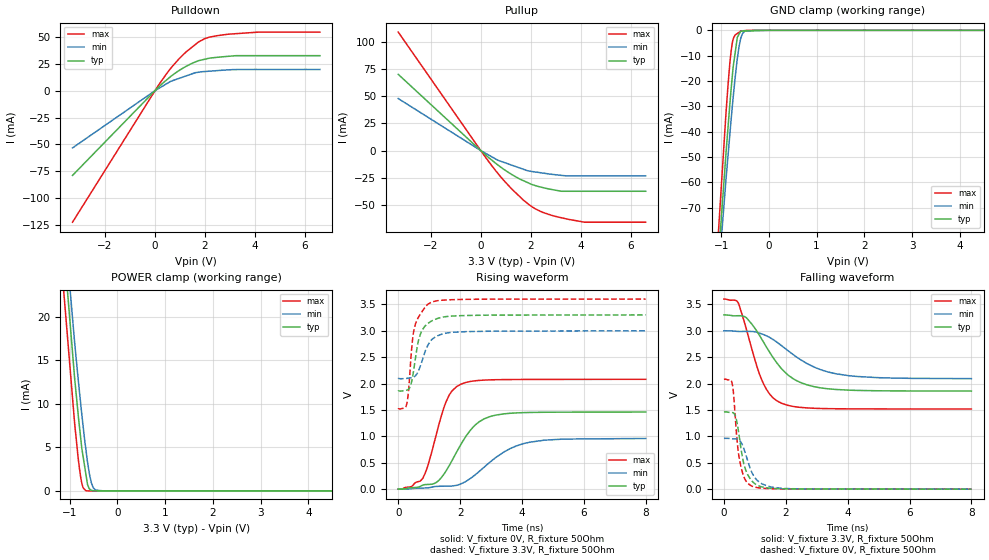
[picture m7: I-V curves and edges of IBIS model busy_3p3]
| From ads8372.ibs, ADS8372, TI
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|   busy_3p3 Model
[Model]   busy_3p3
Model_type   3-state
Polarity   Non-Inverting
Vmeas = 1.65
Vref = 1.65
Cref = 10pF
Rref = 50
|   typ   min   max
|   (nom PVT)   (fast PVT)   (slow PVT)
|C_comp from frequency sweep method (F=1MHz)
|C_comp   3.458e-12   3.339e-12   3.651e-12
|ON state : BUFFER OUTPUT TURNED HIGH
|C_comp   3.458e-12   3.339e-12   3.651e-12
|OFF state: BUFFER IN HIGH IMPEDANCE
|C_comp   2.977e-12   2.823e-12   3.114e-12
|C_comp from LC tank measurement(L=1nH)
|Resonant Frequency(Hz)   5.970e+09   6.100e+09   5.800e+09
|C_comp   7.114e-13   6.814e-13   7.537e-13
|ON state : BUFFER OUTPUT TURNED HIGH
|Resonant Frequency(Hz)   5.970e+09   6.100e+09   5.800e+09
|C_comp   7.114e-13   6.814e-13   7.537e-13
|OFF state: BUFFER IN HIGH IMPEDANCE
|Resonant Frequency(Hz)   6.040e+09   6.210e+09   5.850e+09
C_comp   6.950e-13   6.575e-13   7.409e-13
| Where nom  PVT is Nominal Process, 3.3V, 35C
|   Fast PVT is Strong Process,  3.6V, -40C
|   Slow PVT is Weak Process,   3V, 95C
[Voltage Range]   3.3   3   3.6
|Ambient Temperature   25   85   -40
|Junction Temperature
[Temperature Range]   35   95   -40
[Pullup Reference]   3.3   3   3.6
[Pulldown Reference]   0   0   0
[Power Clamp Reference]   3.3   3   3.6
[GND Clamp Reference]   0   0   0
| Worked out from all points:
|   slope of the pulldown table from 0 to 0.495 V, typ, clamps not added: 46.6 ohm
|   slope of the pullup table from 0 to 0.495 V, typ, clamps not added: 50.7 ohm
|   GND clamp passes 1 mA (typ) near -0.61 V on its own axis
|   POWER clamp passes 1 mA (typ) near -0.63 V on its own axis
|   falling waveform, V_fixture 3.3V, R_fixture 50Ohm: 20-80 % time 1.06ns typ, 1.45ns min, 683ps max; typ from 3.3 V to 1.86 V
|   rising waveform, V_fixture 0V, R_fixture 50Ohm: 20-80 % time 924ps typ, 1.31ns min, 613ps max; typ from 0 V to 1.46 V
|   rising waveform, V_fixture 3.3V, R_fixture 50Ohm: 20-80 % time 304ps typ, 384ps min, 252ps max; typ from 1.86 V to 3.3 V
|   falling waveform, V_fixture 0V, R_fixture 50Ohm: 20-80 % time 304ps typ, 391ps min, 225ps max; typ from 1.46 V to 0.001 V
[Pulldown]
|   Voltage   I(typ)   I(min)   I(max)
-3.3V     -78.98mA   -53.36mA   -122.6mA
176.4mV   4.073mA    2.487mA    6.361mA
633mV     13.32mA    8.781mA    20.94mA
939.6mV   18.45mA    11.28mA    29.19mA
1.246V    22.71mA    13.78mA    36.21mA
1.706V    27.67mA    17.1mA     44.83mA
2.153V    30.2mA     18.15mA    49.79mA
2.934V    32.05mA    19.43mA    52.68mA
4.162V    32.65mA    19.81mA    54.64mA
6.6V      32.65mA    19.81mA    54.64mA
[GND Clamp]
|   Voltage   I(typ)   I(min)   I(max)
-3.3V     -761.3mA   -676.6mA   -965.4mA
-1.115V   -105.4mA   -111.1mA   -97.09mA
-897.6mV  -48.4mA    -58.78mA   -32.56mA
-856.8mV  -38.65mA   -49.79mA   -21.97mA
-792mV    -23.53mA   -35.54mA   -8.421mA
-766.8mV  -18.32mA   -30.35mA   -5.108mA
-738mV    -13.14mA   -24.6mA    -2.94mA
-660mV    -2.733mA   -11.06mA   -1.235mA
-586.8mV  -322.6uA   -3.017mA   -267.8uA
-510mV    -258uA     -378.2uA   -130.5uA
-285mV    -143.4uA   -450.4nA   -1.904uA
6.6V      0A         0A         0A
[Pullup]
|   Voltage   I(typ)   I(min)   I(max)
-3.3V     69.99mA    47.77mA    108.8mA
18mV      -371.7uA   -256.6uA   -591.9uA
478.8mV   -9.46mA    -6.234mA   -15.01mA
708mV     -13.64mA   -9.093mA   -21.59mA
1.246V    -22.07mA   -13.46mA   -35.43mA
1.89V     -29.57mA   -18.59mA   -48.96mA
2.167V    -32.08mA   -19.64mA   -53.36mA
2.473V    -33.96mA   -20.65mA   -56.75mA
2.812V    -35.67mA   -21.75mA   -59.36mA
3.241V    -37.41mA   -22.85mA   -61.83mA
4.151V    -37.41mA   -23.24mA   -65.82mA
6.6V      -37.41mA   -23.24mA   -65.82mA
[POWER Clamp]
|   Voltage   I(typ)   I(min)   I(max)
-3.3V     298.8mA    244.5mA    432.6mA
-1.156V   30.27mA    33.59mA    24.98mA
-897.6mV  13.01mA    17.12mA    7.827mA
-824.4mV  8.877mA    12.96mA    3.87mA
-766.8mV  5.928mA    9.871mA    1.482mA
-720mV    3.976mA    7.457mA    365.5uA
-662.4mV  1.972mA    4.822mA    28.47uA
-627mV    740.4uA    3.325mA    5.896uA
-549mV    64.5uA     984.1uA    3.448uA
-510mV    36.68uA    395.6uA    2.223uA
-462mV    2.437uA    102.5uA    716.8nA
6.6V      0A         0A         0A
[Ramp]
R_load = 50
|   typ   min   max
dV/dt_r   0.876214/9.23938e-10   0.576036/1.31035e-09   1.24786/6.12367e-10
dV/dt_f   0.864611/1.06042e-09   0.543659/1.44481e-09   1.2486/6.81788e-10
[Falling Waveform]
V_fixture = 3.3V
V_fixture_min = 3V
V_fixture_max = 3.6V
R_fixture = 50Ohm
|   Time   V(typ)   V(min)   V(max)
0s        3.3V       3V         3.6V
464ps     3.286V     2.988V     3.528V
724ps     3.249V     2.99V      3.034V
1.02ns    3.032V     2.979V     2.413V
1.228ns   2.836V     2.94V      2.062V
1.518ns   2.556V     2.86V      1.774V
1.86ns    2.283V     2.72V      1.628V
2.444ns   2.029V     2.465V     1.551V
3.62ns    1.889V     2.186V     1.523V
7.998ns   1.859V     2.094V     1.519V
[Rising Waveform]
V_fixture = 0V
V_fixture_min = 0V
V_fixture_max = 0V
R_fixture = 50Ohm
|   Time   V(typ)   V(min)   V(max)
0s        1.371nV    3.229nV    1.196nV
794ps     76.83mV    21.38mV    206.9mV
970ps     89.68mV    25.69mV    469.8mV
1.24ns    131.7mV    52.31mV    1.056V
1.548ns   347.7mV    56.8mV     1.656V
1.744ns   547.3mV    59.32mV    1.864V
2.042ns   864.5mV    104.2mV    1.992V
2.78ns    1.332V     418.4mV    2.066V
4.08ns    1.45V      866.6mV    2.077V
7.998ns   1.46V      960.1mV    2.08V
[Rising Waveform]
V_fixture = 3.3V
V_fixture_min = 3V
V_fixture_max = 3.6V
R_fixture = 50Ohm
|   Time   V(typ)   V(min)   V(max)
0s        1.858V     2.092V     1.519V
282ps     1.876V     2.098V     1.63V
334ps     1.892V     2.103V     1.868V
464ps     2.127V     2.114V     2.84V
554ps     2.471V     2.145V     3.122V
626ps     2.738V     2.206V     3.225V
740ps     2.971V     2.373V     3.338V
1.066ns   3.18V      2.822V     3.539V
2.058ns   3.286V     2.98V      3.593V
7.998ns   3.3V       3V         3.6V
[Falling Waveform]
V_fixture = 0V
V_fixture_min = 0V
V_fixture_max = 0V
R_fixture = 50Ohm
|   Time   V(typ)   V(min)   V(max)
0s        1.461V     961.6mV    2.08V
260ps     1.452V     955.6mV    2.016V
368ps     1.393V     951.8mV    1.353V
438ps     1.213V     947.1mV    842.8mV
506ps     951.7mV    922.9mV    547.8mV
674ps     414.2mV    714.4mV    196.1mV
916ps     147.8mV    301.4mV    55.16mV
1.23ns    42.2mV     100.8mV    17.89mV
1.834ns   8.782mV    17.85mV    5.566mV
7.998ns   517.9uV    609.1uV    198.4uV
